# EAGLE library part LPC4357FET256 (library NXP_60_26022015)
32-bit ARM Cortex-M4/M0 MCU; up to 1 MB flash and 136 kB SRAM; Ethernet, two High-speed USB, LCD, EMC The LPC435x/3x/2x/1x are ARM Cortex-M4 based microcontrollers for embedded applications which include an ARM Cortex-M0 coprocessor, up to 1 MB of flash and 136 kB of on-chip SRAM, 16 kB of EEPROM memory, a quad SPI Flash Interface (SPIFI), advanced configurable peripherals such as the State Configurable Timer (SCT) and the Serial General Purpose I/O (SGPIO) interface, two High-speed USB controllers, Ethernet, LCD, an external memory controller, and multiple digital and analog peripherals. The LPC435x/3x/2x/1x operate at CPU frequencies of up to 204 MHz. The ARM Cortex-M4 is a next generation 32-bit core that offers system enhancements such as low power consumption, enhanced debug features, and a high level of support block integration. The ARM Cortex-M4 CPU incorporates a 3-stage pipeline, uses a Harvard architecture with separate local instruction and data buses as well as a third bus for peripherals, and includes an internal prefetch unit that supports speculative branching. The ARM Cortex-M4 supports single-cycle digital signal processing and SIMD instructions. A hardware floating-point unit is integrated in the core. The ARM Cortex-M0 coprocessor is an energy-efficient and easy-to-use 32-bit core which is upward code- and tool-compatible with the Cortex-M4 core. The Cortex-M0 coprocessor, designed as a replacement for existing 8/16-bit microcontrollers, offers up to 204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
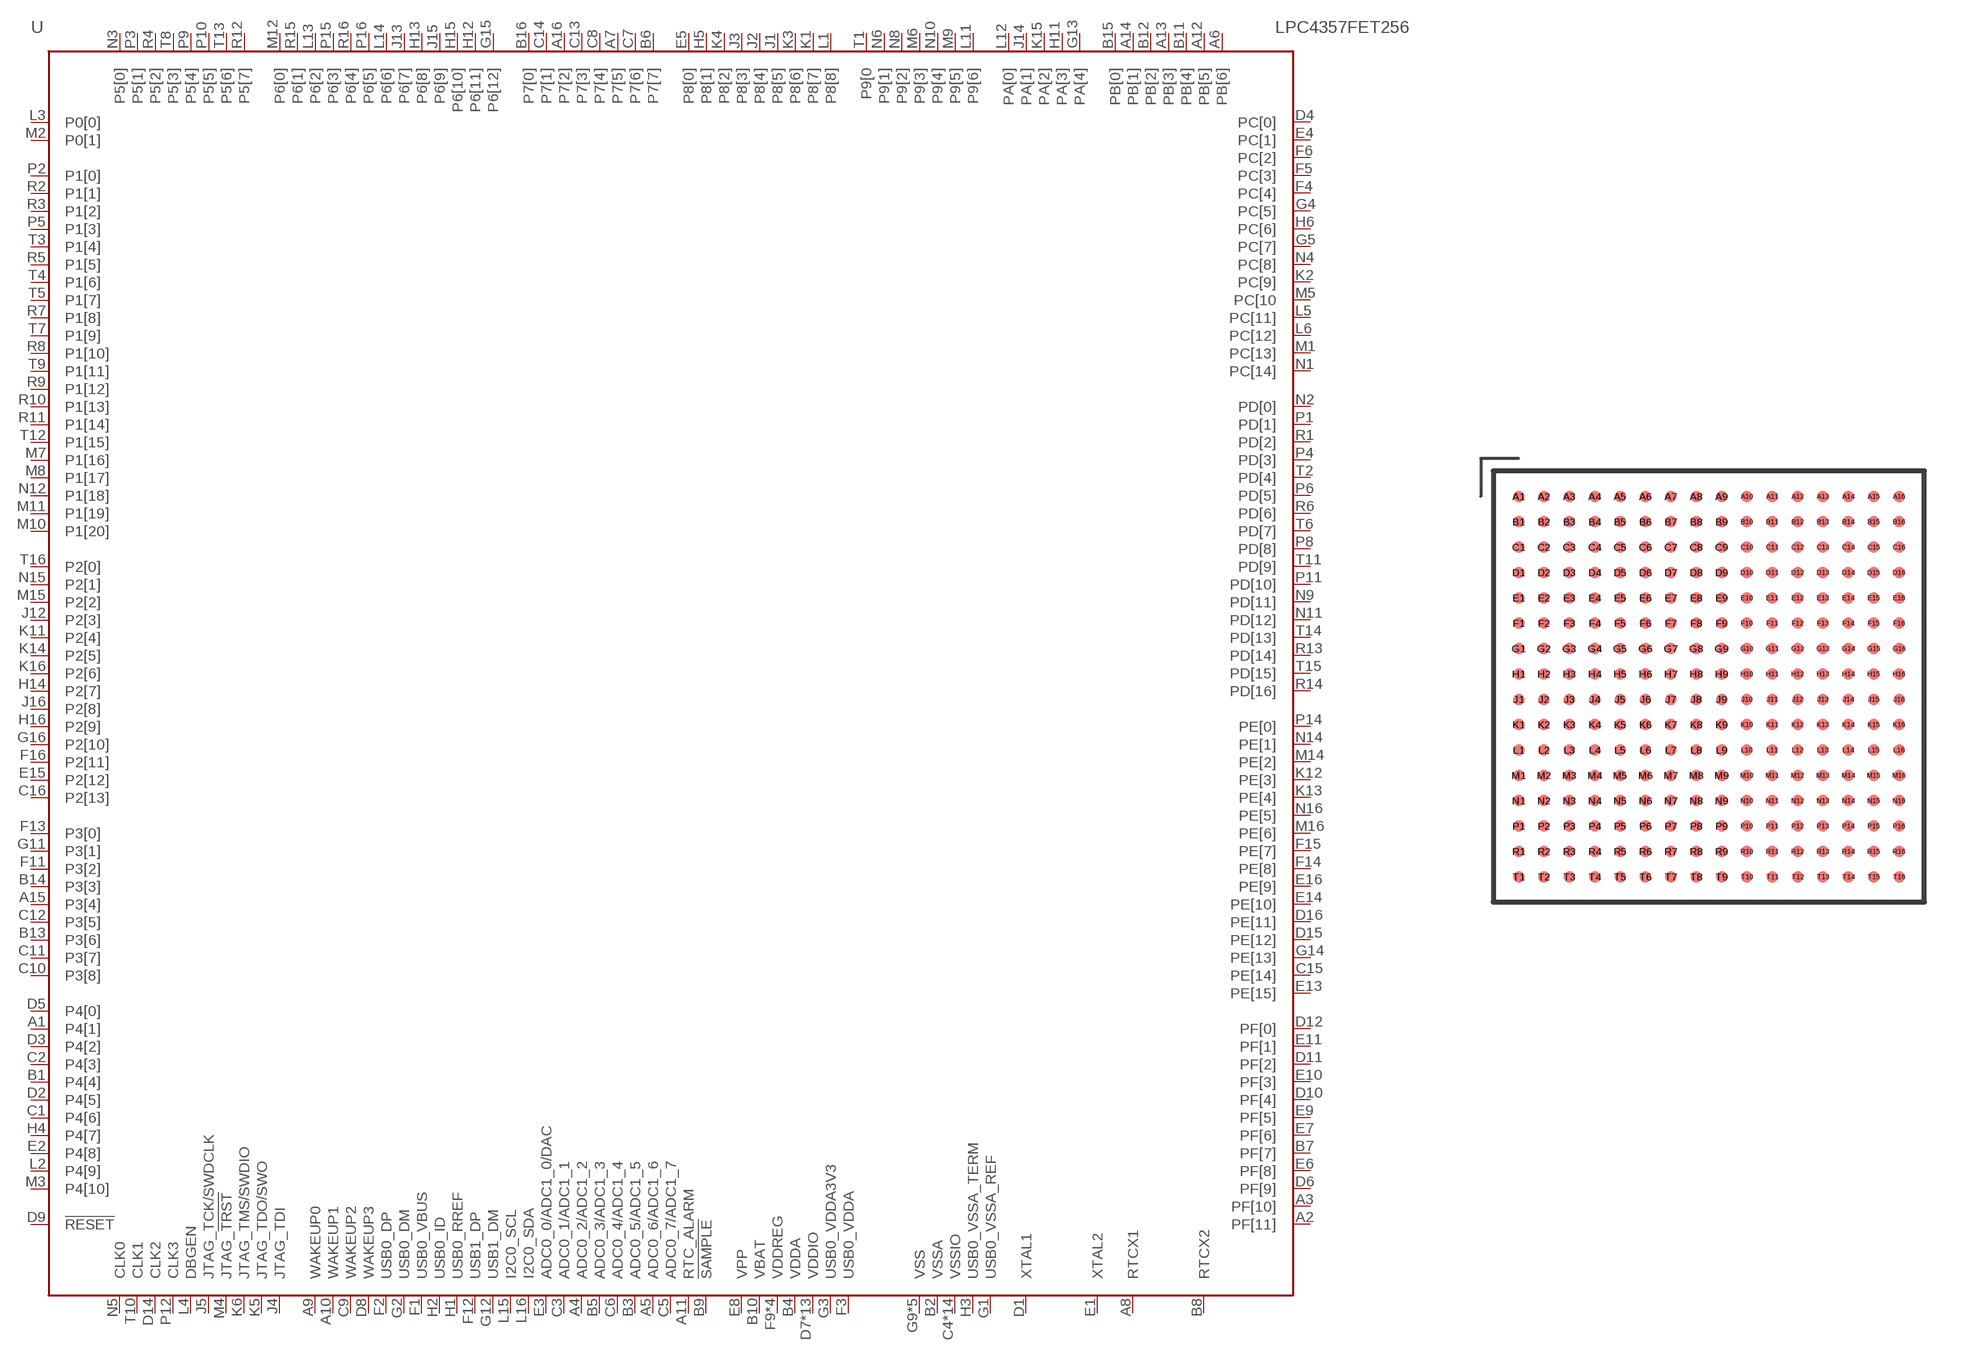
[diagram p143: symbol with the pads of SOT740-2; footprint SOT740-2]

Designator prefix U

## LPC4357FET256  [SOT740-2]
A1  P4[1]
A2  PF[11]
A3  PF[10]
A4  ADC0_2/ADC1_2  in
A5  ADC0_6/ADC1_6  in
A6  PB[6]
A7  P7[5]
A8  RTCX1  in
A9  WAKEUP0  in
A10  WAKEUP1  in
A11  RTC_ALARM  out
A12  PB[5]
A13  PB[3]
A14  PB[1]
A15  P3[4]
A16  P7[2]
B1  P4[4]
B2  VSSA  pwr
B3  ADC0_5/ADC1_5  in
B4  VDDA  pwr
B5  ADC0_3/ADC1_3  in
B6  P7[7]
B7  PF[7]
B8  RTCX2  out
B9  !SAMPLE  out
B10  VBAT  pwr
B11  PB[4]
B12  PB[2]
B13  P3[6]
B14  P3[3]
B15  PB[0]
B16  P7[0]
C1  P4[6]
C2  P4[3]
C3  ADC0_1/ADC1_1  in
C4  VSSIO  pwr
C5  ADC0_7/ADC1_7  in
C6  ADC0_4/ADC1_4  in
C7  P7[6]
C8  P7[4]
C9  WAKEUP2  in
C10  P3[8]
C11  P3[7]
C12  P3[5]
C13  P7[3]
C14  P7[1]
C15  PE[14]
C16  P2[13]
D1  XTAL1  in
D2  P4[5]
D3  P4[2]
D4  PC[0]
D5  P4[0]
D6  PF[9]
D7  VDDIO  pwr
D8  WAKEUP3  in
D9  !RESET!  in
D10  PF[4]
D11  PF[2]
D12  PF[0]
D13  VSSIO  pwr
D14  CLK2
D15  PE[12]
D16  PE[11]
E1  XTAL2  out
E2  P4[8]
E3  ADC0_0/ADC1_0/DAC  in
E4  PC[1]
E5  P8[0]
E6  PF[8]
E7  PF[6]
E8  VPP  pwr
E9  PF[5]
E10  PF[3]
E11  PF[1]
E12  VDDIO  pwr
E13  PE[15]
E14  PE[10]
E15  P2[12]
E16  PE[9]
F1  USB0_VBUS
F2  USB0_DP
F3  USB0_VDDA  pwr
F4  PC[4]
F5  PC[3]
F6  PC[2]
F7  VDDIO  pwr
F8  VDDIO  pwr
F9  VDDREG  pwr
F10  VDDREG  pwr
F11  P3[2]
F12  USB1_DP
F13  P3[0]
F14  PE[8]
F15  PE[7]
F16  P2[11]
G1  USB0_VSSA_REF  pwr
G2  USB0_DM
G3  USB0_VDDA3V3  pwr
G4  PC[5]
G5  PC[7]
G6  VSSIO  pwr
G7  VSSIO  pwr
G8  VSSIO  pwr
G9  VSS  pwr
G10  VDDIO  pwr
G11  P3[1]
G12  USB1_DM
G13  PA[4]
G14  PE[13]
G15  P6[12]
G16  P2[10]
H1  USB0_RREF  pas
H2  USB0_ID  in
H3  USB0_VSSA_TERM  pwr
H4  P4[7]
H5  P8[1]
H6  PC[6]
H7  VSS  pwr
H8  VSSIO  pwr
H9  VSSIO  pwr
H10  VDDIO  pwr
H11  PA[3]
H12  P6[11]
H13  P6[8]
H14  P2[7]
H15  P6[10]
H16  P2[9]
J1  P8[5]
J2  P8[4]
J3  P8[3]
J4  JTAG_TDI  in
J5  JTAG_TCK/SWDCLK  in
J6  VDDIO  pwr
J7  VDDIO  pwr
J8  VSSIO  pwr
J9  VSSIO  pwr
J10  VSS  pwr
J11  VSS  pwr
J12  P2[3]
J13  P6[7]
J14  PA[1]
J15  P6[9]
J16  P2[8]
K1  P8[7]
K2  PC[9]
K3  P8[6]
K4  P8[2]
K5  JTAG_TDO/SWO  out
K6  JTAG_TMS/SWDIO  in
K7  VDDIO  pwr
K8  VSS  pwr
K9  VSSIO  pwr
K10  VSSIO  pwr
K11  P2[4]
K12  PE[3]
K13  PE[4]
K14  P2[5]
K15  PA[2]
K16  P2[6]
L1  P8[8]
L2  P4[9]
L3  P0[0]
L4  DBGEN  in
L5  PC[11]
L6  PC[12]
L7  VDDREG  pwr
L8  VDDREG  pwr
L9  VDDIO  pwr
L10  VDDIO  pwr
L11  P9[6]
L12  PA[0]
L13  P6[2]
L14  P6[6]
L15  I2C0_SCL
L16  I2C0_SDA
M1  PC[13]
M2  P0[1]
M3  P4[10]
M4  JTAG_!TRST  in
M5  PC[10
M6  P9[3]
M7  P1[16]
M8  P1[17]
M9  P9[5]
M10  P1[20]
M11  P1[19]
M12  P6[0]
M13  VSSIO  pwr
M14  PE[2]
M15  P2[2]
M16  PE[6]
N1  PC[14]
N2  PD[0]
N3  P5[0]
N4  PC[8]
N5  CLK0
N6  P9[1]
N7  VDDIO  pwr
N8  P9[2]
N9  PD[11]
N10  P9[4]
N11  PD[12]
N12  P1[18]
N13  VDDIO  pwr
N14  PE[1]
N15  P2[1]
N16  PE[5]
P1  PD[1]
P2  P1[0]
P3  P5[1]
P4  PD[3]
P5  P1[3]
P6  PD[5]
P7  VSSIO  pwr
P8  PD[8]
P9  P5[4]
P10  P5[5]
P11  PD[10]
P12  CLK3
P13  VSSIO  pwr
P14  PE[0]
P15  P6[3]
P16  P6[5]
R1  PD[2]
R2  P1[1]
R3  P1[2]
R4  P5[2]
R5  P1[5]
R6  PD[6]
R7  P1[8]
R8  P1[10]
R9  P1[12]
R10  P1[13]
R11  P1[14]
R12  P5[7]
R13  PD[14]
R14  PD[16]
R15  P6[1]
R16  P6[4]
T1  P9[0
T2  PD[4]
T3  P1[4]
T4  P1[6]
T5  P1[7]
T6  PD[7]
T7  P1[9]
T8  P5[3]
T9  P1[11]
T10  CLK1
T11  PD[9]
T12  P1[15]
T13  P5[6]
T14  PD[13]
T15  PD[15]
T16  P2[0]

## Footprint SOT740-2 (pad centres in mm)
SOT740-2 LBGA256: plastic low profile ball grid array package; 256 balls; body 17 x 17 x 1 mm JEDEC: MO-192 IEC: -- JEITA: --
smd 0.45 x 0.45: A1 -7.5,7.5; A2 -6.5,7.5; A3 -5.5,7.5; A4 -4.5,7.5; A5 -3.5,7.5; A6 -2.5,7.5; A7 -1.5,7.5; A8 -0.5,7.5; A9 0.5,7.5; A10 1.5,7.5; A11 2.5,7.5; A12 3.5,7.5; A13 4.5,7.5; A14 5.5,7.5; A15 6.5,7.5; A16 7.5,7.5; B1 -7.5,6.5; B2 -6.5,6.5; B3 -5.5,6.5; B4 -4.5,6.5; B5 -3.5,6.5; B6 -2.5,6.5; B7 -1.5,6.5; B8 -0.5,6.5; B9 0.5,6.5; B10 1.5,6.5; B11 2.5,6.5; B12 3.5,6.5; B13 4.5,6.5; B14 5.5,6.5; B15 6.5,6.5; B16 7.5,6.5; C1 -7.5,5.5; C2 -6.5,5.5; C3 -5.5,5.5; C4 -4.5,5.5; C5 -3.5,5.5; C6 -2.5,5.5; C7 -1.5,5.5; C8 -0.5,5.5; C9 0.5,5.5; C10 1.5,5.5; C11 2.5,5.5; C12 3.5,5.5; C13 4.5,5.5; C14 5.5,5.5; C15 6.5,5.5; C16 7.5,5.5; D1 -7.5,4.5; D2 -6.5,4.5; D3 -5.5,4.5; D4 -4.5,4.5; D5 -3.5,4.5; D6 -2.5,4.5; D7 -1.5,4.5; D8 -0.5,4.5; D9 0.5,4.5; D10 1.5,4.5; D11 2.5,4.5; D12 3.5,4.5; D13 4.5,4.5; D14 5.5,4.5; D15 6.5,4.5; D16 7.5,4.5; E1 -7.5,3.5; E2 -6.5,3.5; E3 -5.5,3.5; E4 -4.5,3.5; E5 -3.5,3.5; E6 -2.5,3.5; E7 -1.5,3.5; E8 -0.5,3.5; E9 0.5,3.5; E10 1.5,3.5; E11 2.5,3.5; E12 3.5,3.5; E13 4.5,3.5; E14 5.5,3.5; E15 6.5,3.5; E16 7.5,3.5; F1 -7.5,2.5; F2 -6.5,2.5; F3 -5.5,2.5; F4 -4.5,2.5; F5 -3.5,2.5; F6 -2.5,2.5; F7 -1.5,2.5; F8 -0.5,2.5; F9 0.5,2.5; F10 1.5,2.5; F11 2.5,2.5; F12 3.5,2.5; F13 4.5,2.5; F14 5.5,2.5; F15 6.5,2.5; F16 7.5,2.5; G1 -7.5,1.5; G2 -6.5,1.5; G3 -5.5,1.5; G4 -4.5,1.5; G5 -3.5,1.5; G6 -2.5,1.5; G7 -1.5,1.5; G8 -0.5,1.5; G9 0.5,1.5; G10 1.5,1.5; G11 2.5,1.5; G12 3.5,1.5; G13 4.5,1.5; G14 5.5,1.5; G15 6.5,1.5; G16 7.5,1.5; H1 -7.5,0.5; H2 -6.5,0.5; H3 -5.5,0.5; H4 -4.5,0.5; H5 -3.5,0.5; H6 -2.5,0.5; H7 -1.5,0.5; H8 -0.5,0.5; H9 0.5,0.5; H10 1.5,0.5; H11 2.5,0.5; H12 3.5,0.5; H13 4.5,0.5; H14 5.5,0.5; H15 6.5,0.5; H16 7.5,0.5; J1 -7.5,-0.5; J2 -6.5,-0.5; J3 -5.5,-0.5; J4 -4.5,-0.5; J5 -3.5,-0.5; J6 -2.5,-0.5; J7 -1.5,-0.5; J8 -0.5,-0.5; J9 0.5,-0.5; J10 1.5,-0.5; J11 2.5,-0.5; J12 3.5,-0.5; J13 4.5,-0.5; J14 5.5,-0.5; J15 6.5,-0.5; J16 7.5,-0.5; K1 -7.5,-1.5; K2 -6.5,-1.5; K3 -5.5,-1.5; K4 -4.5,-1.5; K5 -3.5,-1.5; K6 -2.5,-1.5; K7 -1.5,-1.5; K8 -0.5,-1.5; K9 0.5,-1.5; K10 1.5,-1.5; K11 2.5,-1.5; K12 3.5,-1.5; K13 4.5,-1.5; K14 5.5,-1.5; K15 6.5,-1.5; K16 7.5,-1.5; L1 -7.5,-2.5; L2 -6.5,-2.5; L3 -5.5,-2.5; L4 -4.5,-2.5; L5 -3.5,-2.5; L6 -2.5,-2.5; L7 -1.5,-2.5; L8 -0.5,-2.5; L9 0.5,-2.5; L10 1.5,-2.5; L11 2.5,-2.5; L12 3.5,-2.5; L13 4.5,-2.5; L14 5.5,-2.5; L15 6.5,-2.5; L16 7.5,-2.5; M1 -7.5,-3.5; M2 -6.5,-3.5; M3 -5.5,-3.5; M4 -4.5,-3.5; M5 -3.5,-3.5; M6 -2.5,-3.5; M7 -1.5,-3.5; M8 -0.5,-3.5; M9 0.5,-3.5; M10 1.5,-3.5; M11 2.5,-3.5; M12 3.5,-3.5; M13 4.5,-3.5; M14 5.5,-3.5; M15 6.5,-3.5; M16 7.5,-3.5; N1 -7.5,-4.5; N2 -6.5,-4.5; N3 -5.5,-4.5; N4 -4.5,-4.5; N5 -3.5,-4.5; N6 -2.5,-4.5; N7 -1.5,-4.5; N8 -0.5,-4.5; N9 0.5,-4.5; N10 1.5,-4.5; N11 2.5,-4.5; N12 3.5,-4.5; N13 4.5,-4.5; N14 5.5,-4.5; N15 6.5,-4.5; N16 7.5,-4.5; P1 -7.5,-5.5; P2 -6.5,-5.5; P3 -5.5,-5.5; P4 -4.5,-5.5; P5 -3.5,-5.5; P6 -2.5,-5.5; P7 -1.5,-5.5; P8 -0.5,-5.5; P9 0.5,-5.5; P10 1.5,-5.5; P11 2.5,-5.5; P12 3.5,-5.5; P13 4.5,-5.5; P14 5.5,-5.5; P15 6.5,-5.5; P16 7.5,-5.5; R1 -7.5,-6.5; R2 -6.5,-6.5; R3 -5.5,-6.5; R4 -4.5,-6.5; R5 -3.5,-6.5; R6 -2.5,-6.5; R7 -1.5,-6.5; R8 -0.5,-6.5; R9 0.5,-6.5; R10 1.5,-6.5; R11 2.5,-6.5; R12 3.5,-6.5; R13 4.5,-6.5; R14 5.5,-6.5; R15 6.5,-6.5; R16 7.5,-6.5; T1 -7.5,-7.5; T2 -6.5,-7.5; T3 -5.5,-7.5; T4 -4.5,-7.5; T5 -3.5,-7.5; T6 -2.5,-7.5; T7 -1.5,-7.5; T8 -0.5,-7.5; T9 0.5,-7.5; T10 1.5,-7.5; T11 2.5,-7.5; T12 3.5,-7.5; T13 4.5,-7.5; T14 5.5,-7.5; T15 6.5,-7.5; T16 7.5,-7.5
